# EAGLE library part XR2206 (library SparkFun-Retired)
XR2206 Monolithic Function Generator
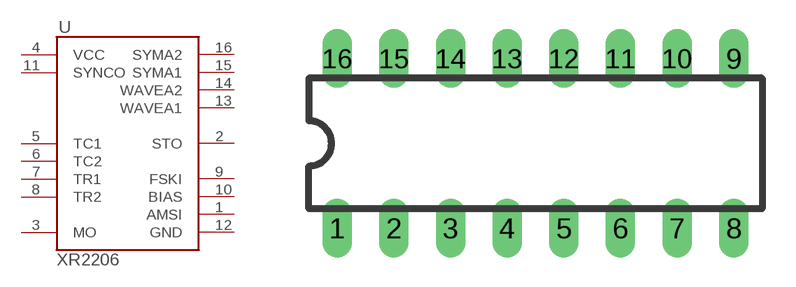
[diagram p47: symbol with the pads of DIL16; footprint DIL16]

Designator prefix U

## XR2206  [DIL16]
1  AMSI  in
2  STO  out
3  MO  out
4  VCC  pwr
5  TC1  in
6  TC2  in
7  TR1  out
8  TR2  out
9  FSKI  in
10  BIAS  out
11  SYNCO  out
12  GND  pwr
13  WAVEA1  in
14  WAVEA2  in
15  SYMA1  in
16  SYMA2  in

## Footprint DIL16 (pad centres in mm)
Dual In Line Package
drill 0.813 long: 1 -8.89,-3.81; 2 -6.35,-3.81; 3 -3.81,-3.81; 4 -1.27,-3.81; 5 1.27,-3.81; 6 3.81,-3.81; 7 6.35,-3.81; 8 8.89,-3.81; 9 8.89,3.81; 10 6.35,3.81; 11 3.81,3.81; 12 1.27,3.81; 13 -1.27,3.81; 14 -3.81,3.81; 15 -6.35,3.81; 16 -8.89,3.81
